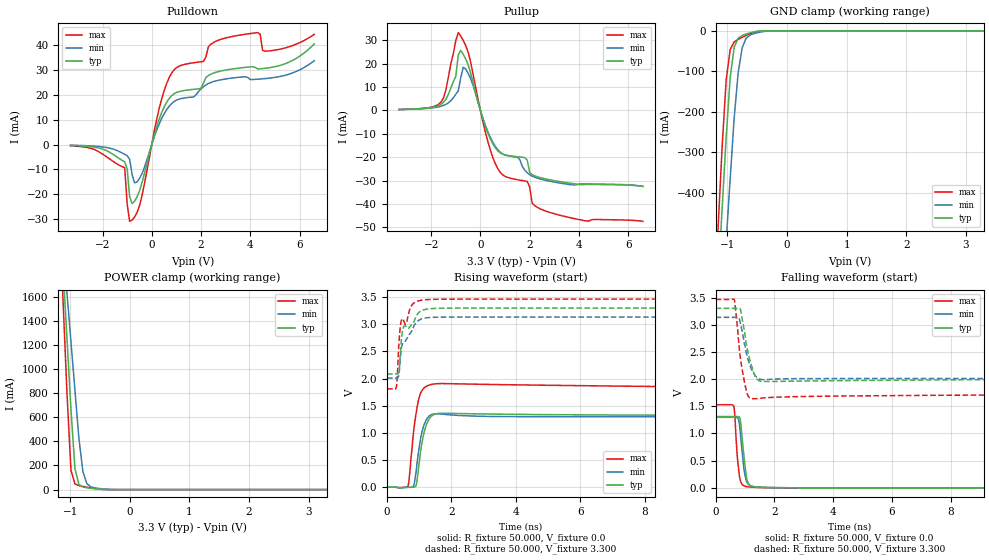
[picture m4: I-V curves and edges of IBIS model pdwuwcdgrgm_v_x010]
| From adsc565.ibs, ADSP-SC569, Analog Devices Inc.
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|   Model pdwuwcdgrgm_v
[Model] pdwuwcdgrgm_v_x010
Model_type I/O
Polarity   Non-Inverting
Enable   Active-Low
Vinl =  0.660V
Vinh =  2.640V
C_comp   1.504pF   1.445pF   1.560pF
C_comp_pullup   0.665pF   0.615pF   0.666pF
C_comp_pulldown   0.430pF   0.388pF   0.445pF
[Model Spec]
Vinh   2.640V   2.508V   2.772V
Vinl   0.660V   0.627V   0.693V
[Temperature Range]   25.000   0.125k   -40.000
[Voltage Range]   3.300V   3.135V   3.465V
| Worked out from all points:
|   slope of the pulldown table from 0 to 0.495 V, typ, clamps not added: 33.1 ohm
|   slope of the pullup table from 0 to 0.495 V, typ, clamps not added: 35.2 ohm
|   GND clamp passes 1 mA (typ) near -0.49 V on its own axis
|   POWER clamp passes 1 mA (typ) near -0.44 V on its own axis
|   rising waveform, R_fixture 50.000, V_fixture 0.0: 20-80 % time 209ps typ, 198ps min, 162ps max; typ from 0 V to 1.31 V
|   rising waveform, R_fixture 50.000, V_fixture 3.300: 20-80 % time 445ps typ, 394ps min, 317ps max; typ from 2.09 V to 3.3 V
|   falling waveform, R_fixture 50.000, V_fixture 0.0: 20-80 % time 155ps typ, 155ps min, 124ps max; typ from 1.31 V to 0 V
|   falling waveform, R_fixture 50.000, V_fixture 3.300: 20-80 % time 257ps typ, 288ps min, 211ps max; typ from 3.3 V to 2.08 V
[Pulldown]
|Voltage   I(typ)   I(min)   I(max)
-3.3V     -393.2uA   -287.2uA   -539.1uA
-1.1V     -7mA       -3.96mA    -9.323mA
-1V       -9.726mA   -4.467mA   -23.88mA
-900mV    -20.95mA   -5.949mA   -30.91mA
-600mV    -21.14mA   -15.07mA   -27.41mA
300mV     10.17mA    8.237mA    14.46mA
900mV     20.4mA     17.24mA    30.02mA
2.1V      24.74mA    23.26mA    33.46mA
3V        29.96mA    26.38mA    42.88mA
4.3V      30.41mA    26.28mA    45.06mA
4.6V      30.67mA    26.53mA    37.58mA
6.6V      40.48mA    33.73mA    44.35mA
[Pullup]
|Voltage   I(typ)   I(min)   I(max)
-3.3V     405.9uA    368.3uA    387.8uA
-1.6V     2.638mA    1.779mA    3.558mA
-1V       14.55mA    6.887mA    29.77mA
-900mV    23.66mA    8.334mA    33.27mA
-700mV    24.05mA    18.42mA    29.96mA
-600mV    22.06mA    17.71mA    27.76mA
300mV     -9.598mA   -9.048mA   -13.22mA
900mV     -18.67mA   -18.58mA   -27.48mA
1.9V      -21.17mA   -26.6mA    -30.35mA
2.1V      -27.43mA   -28.09mA   -39.6mA
2.7V      -29.4mA    -29.99mA   -43.19mA
6.6V      -32.46mA   -32.47mA   -47.38mA
[GND_clamp]
|Voltage   I(typ)   I(min)   I(max)
-3.3V     -6.331A    -5.928A    -6.883A
-1.156V   -612.4mA   -832mA     -480.5mA
-1.089V   -436.3mA   -675.2mA   -283.9mA
-1.022V   -261.8mA   -519.3mA   -121mA
-955mV    -115.5mA   -364.6mA   -46.32mA
-888mV    -40.48mA   -215.6mA   -27.35mA
-821mV    -18.03mA   -103.2mA   -21.08mA
-754mV    -11.67mA   -42.19mA   -16.02mA
-687mV    -7.883mA   -18.25mA   -11.37mA
-620mV    -4.816mA   -10.3mA    -7.232mA
-352mV    -29.83uA   -1.015mA   -30.22uA
3.3V      0A         0A         0A
[POWER_clamp]
|Voltage   I(typ)   I(min)   I(max)
-3.3V     21.2A      15.36A     27.27A
-1.189V   2.436A     2.445A     2.368A
-1.122V   1.844A     2.038A     1.583A
-1.055V   1.254A     1.632A     800mA
-988mV    665.4mA    1.226A     161.7mA
-921mV    175.4mA    823mA      47.01mA
-854mV    42.66mA    422.6mA    32.46mA
-787mV    21.34mA    146.7mA    25.7mA
-720mV    15.03mA    48.63mA    19.66mA
-653mV    10.52mA    22.18mA    14.07mA
-251mV    4.083uA    411.3uA    1.265uA
3.3V      0A         0A         0A
[Ramp]
| variable   typ   min   max
dV/dt_r   0.786/0.208n   0.778/0.199n   0.940/0.161n
dV/dt_f   0.730/0.257n   0.675/0.291n   1.003/0.214n
R_load = 50.000
[Rising Waveform]
R_fixture= 50.000
V_fixture= 0.0
V_fixture_min= 0.0
V_fixture_max= 0.0
|time   V(typ)   V(min)   V(max)
0s        279.7nV    106.4uV    162.3nV
650ps     -2.627mV   -2.558mV   18.88mV
690ps     -2.072mV   -1.878mV   158.3mV
840ps     111.9uV    48.8mV     1.092V
920ps     72.02mV    369.3mV    1.413V
1.03ns    600.9mV    840.2mV    1.712V
1.23ns    1.165V     1.25V      1.862V
1.62ns    1.36V      1.351V     1.908V
45.97ns   1.311V     1.297V     1.676V
100ns     1.311V     1.297V     1.566V
[Rising Waveform]
R_fixture= 50.000
V_fixture= 3.300
V_fixture_min= 3.135
V_fixture_max= 3.465
|time   V(typ)   V(min)   V(max)
0s        2.086V     2.011V     1.812V
290ps     2.086V     2.01V      1.84V
320ps     2.085V     2.01V      2.032V
370ps     2.135V     2.082V     2.637V
460ps     2.783V     2.594V     3.093V
590ps     2.957V     2.712V     3.005V
730ps     2.968V     2.84V      3.317V
940ps     3.18V      3.053V     3.425V
1.44ns    3.293V     3.13V      3.461V
100ns     3.3V       3.135V     3.465V
[Falling Waveform]
R_fixture= 50.000
V_fixture= 0.0
V_fixture_min= 0.0
V_fixture_max= 0.0
|time   V(typ)   V(min)   V(max)
0s        1.311V     1.297V     1.529V
620ps     1.311V     1.298V     1.496V
660ps     1.311V     1.298V     1.286V
740ps     1.312V     1.289V     570.3mV
810ps     1.302V     1.167V     225.4mV
860ps     1.167V     898.5mV    107.5mV
960ps     611.2mV    366.8mV    37.91mV
1.08ns    127.5mV    95.74mV    20.65mV
1.52ns    12.21mV    12.61mV    6.196mV
100ns     5.101uV    106.1uV    5.304uV
[Falling Waveform]
R_fixture= 50.000
V_fixture= 3.300
V_fixture_min= 3.135
V_fixture_max= 3.465
|time   V(typ)   V(min)   V(max)
0s        3.3V       3.135V     3.465V
640ps     3.3V       3.135V     3.455V
780ps     3.302V     3.136V     2.717V
840ps     3.289V     3.038V     2.405V
990ps     2.86V      2.627V     1.917V
1.12ns    2.445V     2.337V     1.678V
1.29ns    2.125V     2.111V     1.639V
1.46ns    1.977V     2.011V     1.645V
1.76ns    1.956V     1.992V     1.659V
100ns     2.084V     2.011V     1.793V
